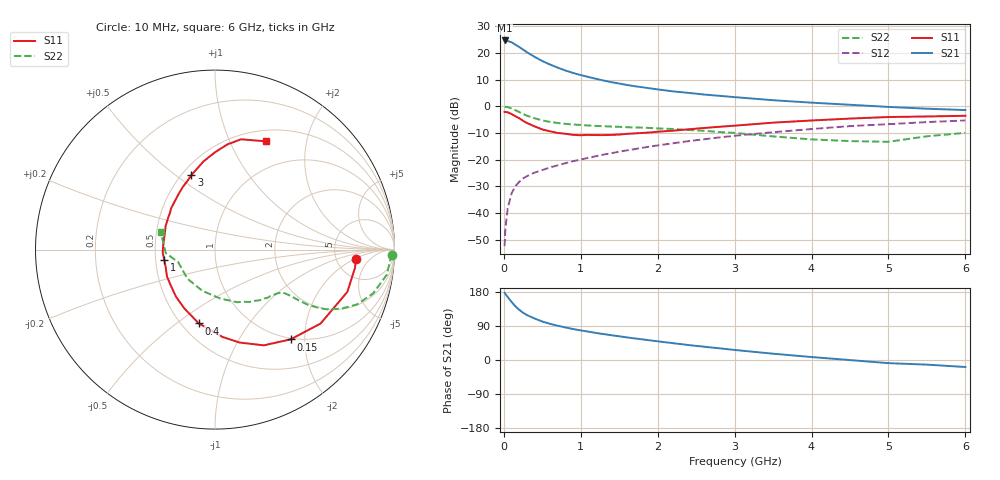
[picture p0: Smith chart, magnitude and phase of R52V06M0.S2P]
! SIEMENS Small Signal Semiconductors
! BFR183
! Si NPN RF Bipolar Junction Transistor in SOT23
! VCE = 2 V  IC = 6 mA
! Common Emitter S-Parameters:  May  1996
# GHz  S  MA  R  50
!  f  S11  S21  S12  S22
! GHz  MAG  ANG  MAG  ANG  MAG  ANG  MAG  ANG
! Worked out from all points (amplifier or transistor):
!   36 points, 10 MHz to 6 GHz, reference 50 ohm
!   highest |S21| = 24.7 dB at 10 MHz (marker M1)
!   |S21| within 3 dB of that: start of sweep to 228.3 MHz
!   unconditionally stable (mu >= 1): 936.4 MHz to 2.623 GHz
!   at 250 MHz: K = 0.48, MSG = 24.2 dB, |S12| = -27.0 dB
!   at 1.4 GHz: K = 1.07, MAG = 11.7 dB, |S12| = -17.5 dB
!   at 6 GHz: K = 0.89, MSG = 1.9 dB, |S12| = -5.3 dB
!   lowest NFmin = 1.20 dB at 450 MHz
!   S11 on the Smith chart (normalised r, x): 10 MHz: 7.82, -2.09; 150 MHz: 0.98, -1.71; 400 MHz: 0.61, -0.61; 1 GHz: 0.56, -0.07; 3 GHz: 0.56, +0.57; 6 GHz: 0.63, +1.37
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0.01  0.787 -3.7  17.18 177.3  0.0024 86.5  0.9889 -1.6
0.02  0.7866 -7.4  17.05 174.2  0.0052 89.5  0.9784 -3.3
0.05  0.7741 -17.7  16.78 166.2  0.0122 80.6  0.9678 -8.3
0.1  0.7182 -35.0  15.89 153.4  0.0233 73.3  0.914 -15.5
0.15  0.654 -49.9  14.31 141.7  0.032 67.0  0.8484 -21.1
0.2  0.5987 -63.0  12.95 132.5  0.0386 63.3  0.7816 -24.8
0.25  0.5351 -75.3  11.59 124.7  0.0445 59.8  0.7192 -27.7
0.3  0.4881 -85.2  10.34 118.6  0.0493 58.8  0.6692 -29.2
0.4  0.4213 -102.3  8.464 109.5  0.0573 56.8  0.5979 -30.8
0.5  0.3698 -117.5  7.063 101.5  0.0641 56.9  0.5456 -31.2
0.6  0.3406 -129.7  6.083 95.6  0.0716 57.4  0.5112 -31.4
0.8  0.3068 -150.7  4.698 85.9  0.0861 58.3  0.47 -31.8
1  0.2882 -168.5  3.86 78.1  0.1009 59.5  0.4477 -32.6
1.1  0.2921 -176.8  3.548 74.7  0.1088 59.8  0.4387 -33.5
1.3  0.2895 170.7  3.039 68.3  0.1252 60.1  0.4238 -35.2
1.6  0.3053 154.2  2.514 59.6  0.1499 59.5  0.4065 -38.9
2.2  0.3498 130.0  1.909 44.4  0.2034 56.7  0.3767 -48.5
3  0.4346 107.7  1.489 26.5  0.281 49.4  0.318 -67.2
3.5  0.4952 97.5  1.304 16.6  0.3278 43.7  0.2738 -84.0
4.5  0.5901 83.3  1.071 -0.2  0.4263 31.4  0.2234 -133.5
5.5  0.6463 70.3  0.904 -12.2  0.5076 19.1  0.275 -175.9
6  0.6662 65.0  0.852 -18.5  0.545 11.0  0.3191 161.8
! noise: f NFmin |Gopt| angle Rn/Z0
0.45  1.2  0.21  41  0.24
0.9  1.25  0.24  101  0.21
1.8  2  0.32  175  0.14
